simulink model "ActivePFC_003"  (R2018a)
settings: Solver=FixedStepDiscrete  StartTime=0.0  StopTime=inf  RelTol=1e-3  EnableMultiTasking=on
model workspace (MAT data in the model file):
  VoRef = 700
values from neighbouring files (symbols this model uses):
  Tcontrol = 5e-5    (= 5e-05)    [Sample_Time.m]
  Tmeasure = 5e-5     *2    (= 0.0001)    [Sample_Time.m]
  Tsample = 1e-6    (= 1e-06)    [Sample_Time.m]
  Tscope = Tcontrol*20    (= 0.001)    [Sample_Time.m]
undefined symbols (not defined in the file or in its folder): A, ADCIN0, ADCIN1, ADCINA0, ADCINB0, bit, Compare, Control, controller, conversion, DCAEVT1, DCAEVT1FILT, Digital, DiscIntNeverNeededParam, ended, Event, Filtered, GPTRIP1SEL, GPTRIP2SEL, input, Module, of, PI, PWM_Library, Single, start, Trip, TZ1, TZ2, version, Zone
libraries: c2837xDlib x23, c2802xlib x5, simulink x3, simulink_extras x2

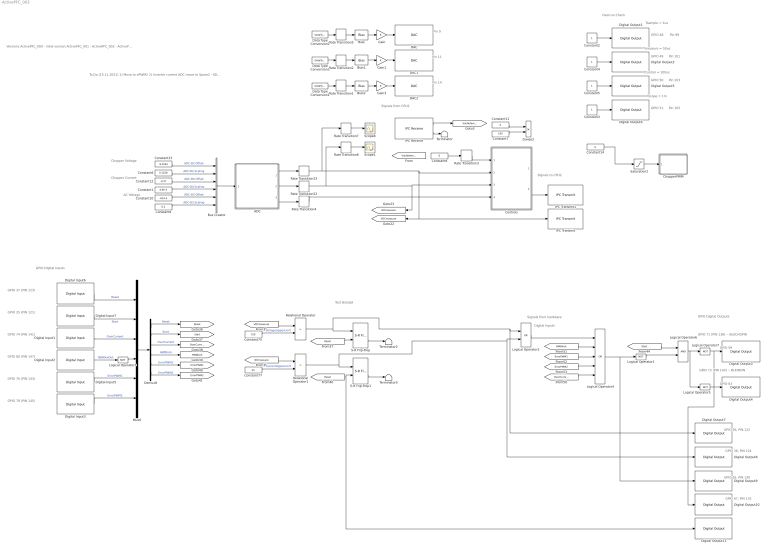
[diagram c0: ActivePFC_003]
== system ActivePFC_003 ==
  note: Test Bistabil
  note: GPIO 38, PIN 124
  note: GPIO 36, PIN 122
  note: GPIO 35 (PIN 121)
  note: GPIO 59
  note: GPIO 63
  note: GPIO Digital Inputs
  note: Digital Inputs
  note: GPIO 74 (PIN 141)
  note: GPIO Digital Outputs
  note: GPIO 80 (PIN 147)
  note: GPIO 37 (PIN 123)
  note: GPIO 78 (PIN 145)
  note: Signals to CPU2
  note: GPIO 73 (PIN 140) -- BLKINVIN
  note: GPIO 76 (PIN 143)
  note: GPIO 71 (PIN 138) -- BLKCHOPIN
  note: Signals from hardware
  note: GPIO 49
  note: Overrun Check
  note: Tcontrol = 100us
  note: Pin 105
  note: Pin 99
  note: Tmeasure = 50us
  note: GPIO 50
  note: GPIO 48
  note: Pin 101
  note: GPIO 51
  note: Pin 103
  note: Tsample = 1us
  note: Tscope = 1m
  note: GPIO 67, PIN 132
  note: GPIO 65, PIN 130
  note: Chopper Current
  note: AC Voltage
  note: Chopper Voltage
  note: Pin 11
  note: Pin 14
  note: Pin 9
  note: Versions ActivePFC_000 - inital version ActivePFC_001 - ActivePFC_002 - ActivePFC_003 - current version ActivePFC_004 - future version
  note: To Do (15.11.2021) 1) Move to ePWM2 2) Inverter current ADC move to Spare2 - ADC-B5 (Pin 26) 3) Change PCB resistor to 100 Ohm for Spare2 4) Check scaling for Spare2
  note: Signals from CPU2
  ADC : Subsystem
  Bias : Bias  Commented=on  Bias=0.0
  Bias1 : Bias  Commented=on  Bias=0.0
  Bias2 : Bias  Commented=on  Bias=0.0
  Bus Creator : BusCreator  Inputs=6
  ChopperPWM : Subsystem
  Constant1 : Constant  Value=4.9e-3  OutDataTypeStr=single  SampleTime=0.1
  Constant10 : Constant  Value=-614.4  OutDataTypeStr=single  SampleTime=0.1
  Constant11 : Constant  Value=0  OutDataTypeStr=single  SampleTime=Tcontrol
  Constant12 : Constant  Value=-0.27  OutDataTypeStr=single  SampleTime=0.1
  Constant13 : Constant  Value=-9.2581  OutDataTypeStr=single  SampleTime=0.1
  Constant14 : Constant  Value=0  OutDataTypeStr=single  SampleTime=Tcontrol
  Constant2 : Constant  Commented=on  SampleTime=Tsample
  Constant3 : Constant  SampleTime=Tscope
  Constant4 : Constant  SampleTime=Tmeasure
  Constant5 : Constant  SampleTime=Tcontrol
  Constant6 : Constant  Value=0.1228  OutDataTypeStr=single  SampleTime=0.1
  Constant7 : Constant  Value=100  OutDataTypeStr=single  SampleTime=Tcontrol
  Constant75 : Constant  Value=750  OutDataTypeStr=single  SampleTime=Tcontrol
  Constant77 : Constant  Value=20  OutDataTypeStr=single  SampleTime=Tcontrol
  Constant8 : Constant  Value=0  OutDataTypeStr=single  SampleTime=Tcontrol
  Constant9 : Constant  Value=0.3  OutDataTypeStr=single  SampleTime=0.1
  Controls : Subsystem
  DAC : c2837xDlib/DAC  Commented=on  channel=A  saturate=off
  DAC1 : c2837xDlib/DAC  Commented=on  channel=B  saturate=off
  DAC2 : c2837xDlib/DAC  Commented=on  channel=C  saturate=off
  Data Type Conversion1 : DataTypeConversion  Commented=on  OutDataTypeStr=single
  Data Type Conversion2 : DataTypeConversion  Commented=on  OutDataTypeStr=single
  Data Type Conversion3 : DataTypeConversion  Commented=on  OutDataTypeStr=single
  Demux8 : Demux  Outputs=6
  Digital Input1 : c2837xDlib/Digital Input  GPIO_Number=GPIO72~GPIO79  GPIO_Bit0=off  GPIO_Bit1=off  GPIO_Bit2=on  GPIO_Bit3=off  GPIO_Bit4=off  GPIO_Bit5=off  GPIO_Bit6=off  GPIO_Bit7=off  sampleTime=Tcontrol  dataType=auto  GPIO_Bit0_Qualification=Sync to SYSCLKOUT  GPIO_Bit1_Qualification=Sync to SYSCLKOUT  GPIO_Bit2_Qualification=Sync to SYSCLKOUT  GPIO_Bit3_Qualification=Sync to SYSCLKOUT  GPIO_Bit4_Qualification=Sync to SYSCLKOUT  GPIO_Bit5_Qualification=Sync to SYSCLKOUT  GPIO_Bit6_Qualification=Sync to SYSCLKOUT  GPIO_Bit7_Qualification=Sync to SYSCLKOUT  Qualification_Period=-1
  Digital Input2 : c2837xDlib/Digital Input  GPIO_Number=GPIO80~GPIO87  GPIO_Bit0=on  GPIO_Bit1=off  GPIO_Bit2=off  GPIO_Bit3=off  GPIO_Bit4=off  GPIO_Bit5=off  GPIO_Bit6=off  GPIO_Bit7=off  sampleTime=Tcontrol  dataType=auto  GPIO_Bit0_Qualification=Sync to SYSCLKOUT  GPIO_Bit1_Qualification=Sync to SYSCLKOUT  GPIO_Bit2_Qualification=Sync to SYSCLKOUT  GPIO_Bit3_Qualification=Sync to SYSCLKOUT  GPIO_Bit4_Qualification=Sync to SYSCLKOUT  GPIO_Bit5_Qualification=Sync to SYSCLKOUT  GPIO_Bit6_Qualification=Sync to SYSCLKOUT  GPIO_Bit7_Qualification=Sync to SYSCLKOUT  Qualification_Period=-1
  Digital Input3 : c2837xDlib/Digital Input  GPIO_Number=GPIO72~GPIO79  GPIO_Bit0=off  GPIO_Bit1=off  GPIO_Bit2=off  GPIO_Bit3=off  GPIO_Bit4=off  GPIO_Bit5=off  GPIO_Bit6=on  GPIO_Bit7=off  sampleTime=Tcontrol  dataType=auto  GPIO_Bit0_Qualification=Sync to SYSCLKOUT  GPIO_Bit1_Qualification=Sync to SYSCLKOUT  GPIO_Bit2_Qualification=Sync to SYSCLKOUT  GPIO_Bit3_Qualification=Sync to SYSCLKOUT  GPIO_Bit4_Qualification=Sync to SYSCLKOUT  GPIO_Bit5_Qualification=Sync to SYSCLKOUT  GPIO_Bit6_Qualification=Sync to SYSCLKOUT  GPIO_Bit7_Qualification=Sync to SYSCLKOUT  Qualification_Period=-1
  Digital Input5 : c2837xDlib/Digital Input  GPIO_Number=GPIO72~GPIO79  GPIO_Bit0=off  GPIO_Bit1=off  GPIO_Bit2=off  GPIO_Bit3=off  GPIO_Bit4=on  GPIO_Bit5=off  GPIO_Bit6=off  GPIO_Bit7=off  sampleTime=Tcontrol  dataType=auto  GPIO_Bit0_Qualification=Sync to SYSCLKOUT  GPIO_Bit1_Qualification=Sync to SYSCLKOUT  GPIO_Bit2_Qualification=Sync to SYSCLKOUT  GPIO_Bit3_Qualification=Sync to SYSCLKOUT  GPIO_Bit4_Qualification=Sync to SYSCLKOUT  GPIO_Bit5_Qualification=Sync to SYSCLKOUT  GPIO_Bit6_Qualification=Sync to SYSCLKOUT  GPIO_Bit7_Qualification=Sync to SYSCLKOUT  Qualification_Period=-1
  Digital Input6 : c2837xDlib/Digital Input  GPIO_Number=GPIO32~GPIO39  GPIO_Bit0=off  GPIO_Bit1=off  GPIO_Bit2=off  GPIO_Bit3=off  GPIO_Bit4=off  GPIO_Bit5=on  GPIO_Bit6=off  GPIO_Bit7=off  sampleTime=Tcontrol  dataType=auto  GPIO_Bit0_Qualification=Sync to SYSCLKOUT  GPIO_Bit1_Qualification=Sync to SYSCLKOUT  GPIO_Bit2_Qualification=Sync to SYSCLKOUT  GPIO_Bit3_Qualification=Sync to SYSCLKOUT  GPIO_Bit4_Qualification=Sync to SYSCLKOUT  GPIO_Bit5_Qualification=Sync to SYSCLKOUT  GPIO_Bit6_Qualification=Sync to SYSCLKOUT  GPIO_Bit7_Qualification=Sync to SYSCLKOUT  Qualification_Period=-1
  Digital Input7 : c2837xDlib/Digital Input  GPIO_Number=GPIO32~GPIO39  GPIO_Bit0=off  GPIO_Bit1=off  GPIO_Bit2=off  GPIO_Bit3=on  GPIO_Bit4=off  GPIO_Bit5=off  GPIO_Bit6=off  GPIO_Bit7=off  sampleTime=Tcontrol  dataType=auto  GPIO_Bit0_Qualification=Sync to SYSCLKOUT  GPIO_Bit1_Qualification=Sync to SYSCLKOUT  GPIO_Bit2_Qualification=Sync to SYSCLKOUT  GPIO_Bit3_Qualification=Sync to SYSCLKOUT  GPIO_Bit4_Qualification=Sync to SYSCLKOUT  GPIO_Bit5_Qualification=Sync to SYSCLKOUT  GPIO_Bit6_Qualification=Sync to SYSCLKOUT  GPIO_Bit7_Qualification=Sync to SYSCLKOUT  Qualification_Period=-1
  Digital Output1 : c2837xDlib/Digital Output  Commented=on  GPIO_Number=GPIO48~GPIO55  GPIO_Bit0=on  GPIO_BIT0_Toggle=on  GPIO_Bit1=off  GPIO_BIT1_Toggle=off  GPIO_Bit2=off  GPIO_BIT2_Toggle=on  GPIO_Bit3=off  GPIO_BIT3_Toggle=off  GPIO_Bit4=off  GPIO_BIT4_Toggle=off  GPIO_Bit5=off  GPIO_BIT5_Toggle=off  GPIO_Bit6=off  GPIO_BIT6_Toggle=off  GPIO_Bit7=off  GPIO_BIT7_Toggle=off
  Digital Output10 : c2837xDlib/Digital Output  GPIO_Number=GPIO64~GPIO71  GPIO_Bit0=off  GPIO_BIT0_Toggle=off  GPIO_Bit1=off  GPIO_BIT1_Toggle=off  GPIO_Bit2=off  GPIO_BIT2_Toggle=off  GPIO_Bit3=on  GPIO_BIT3_Toggle=off  GPIO_Bit4=off  GPIO_BIT4_Toggle=off  GPIO_Bit5=off  GPIO_BIT5_Toggle=off  GPIO_Bit6=off  GPIO_BIT6_Toggle=off  GPIO_Bit7=off  GPIO_BIT7_Toggle=off
  Digital Output11 : c2837xDlib/Digital Output  GPIO_Number=GPIO64~GPIO71  GPIO_Bit0=off  GPIO_BIT0_Toggle=off  GPIO_Bit1=off  GPIO_BIT1_Toggle=off  GPIO_Bit2=off  GPIO_BIT2_Toggle=off  GPIO_Bit3=off  GPIO_BIT3_Toggle=off  GPIO_Bit4=off  GPIO_BIT4_Toggle=off  GPIO_Bit5=on  GPIO_BIT5_Toggle=off  GPIO_Bit6=off  GPIO_BIT6_Toggle=off  GPIO_Bit7=off  GPIO_BIT7_Toggle=off
  Digital Output2 : c2837xDlib/Digital Output  GPIO_Number=GPIO48~GPIO55  GPIO_Bit0=off  GPIO_BIT0_Toggle=on  GPIO_Bit1=on  GPIO_BIT1_Toggle=on  GPIO_Bit2=off  GPIO_BIT2_Toggle=on  GPIO_Bit3=off  GPIO_BIT3_Toggle=off  GPIO_Bit4=off  GPIO_BIT4_Toggle=off  GPIO_Bit5=off  GPIO_BIT5_Toggle=off  GPIO_Bit6=off  GPIO_BIT6_Toggle=off  GPIO_Bit7=off  GPIO_BIT7_Toggle=off
  Digital Output3 : c2837xDlib/Digital Output  GPIO_Number=GPIO64~GPIO71  GPIO_Bit0=off  GPIO_BIT0_Toggle=off  GPIO_Bit1=off  GPIO_BIT1_Toggle=off  GPIO_Bit2=off  GPIO_BIT2_Toggle=off  GPIO_Bit3=off  GPIO_BIT3_Toggle=off  GPIO_Bit4=off  GPIO_BIT4_Toggle=off  GPIO_Bit5=off  GPIO_BIT5_Toggle=off  GPIO_Bit6=off  GPIO_BIT6_Toggle=off  GPIO_Bit7=on  GPIO_BIT7_Toggle=off
  Digital Output4 : c2837xDlib/Digital Output  GPIO_Number=GPIO72~GPIO79  GPIO_Bit0=off  GPIO_BIT0_Toggle=off  GPIO_Bit1=on  GPIO_BIT1_Toggle=off  GPIO_Bit2=off  GPIO_BIT2_Toggle=off  GPIO_Bit3=off  GPIO_BIT3_Toggle=off  GPIO_Bit4=off  GPIO_BIT4_Toggle=off  GPIO_Bit5=off  GPIO_BIT5_Toggle=off  GPIO_Bit6=off  GPIO_BIT6_Toggle=off  GPIO_Bit7=off  GPIO_BIT7_Toggle=off
  Digital Output5 : c2837xDlib/Digital Output  GPIO_Number=GPIO48~GPIO55  GPIO_Bit0=off  GPIO_BIT0_Toggle=off  GPIO_Bit1=off  GPIO_BIT1_Toggle=off  GPIO_Bit2=on  GPIO_BIT2_Toggle=on  GPIO_Bit3=off  GPIO_BIT3_Toggle=off  GPIO_Bit4=off  GPIO_BIT4_Toggle=off  GPIO_Bit5=off  GPIO_BIT5_Toggle=off  GPIO_Bit6=off  GPIO_BIT6_Toggle=off  GPIO_Bit7=off  GPIO_BIT7_Toggle=off
  Digital Output6 : c2837xDlib/Digital Output  GPIO_Number=GPIO48~GPIO55  GPIO_Bit0=off  GPIO_BIT0_Toggle=on  GPIO_Bit1=off  GPIO_BIT1_Toggle=off  GPIO_Bit2=off  GPIO_BIT2_Toggle=on  GPIO_Bit3=on  GPIO_BIT3_Toggle=on  GPIO_Bit4=off  GPIO_BIT4_Toggle=off  GPIO_Bit5=off  GPIO_BIT5_Toggle=off  GPIO_Bit6=off  GPIO_BIT6_Toggle=off  GPIO_Bit7=off  GPIO_BIT7_Toggle=off
  Digital Output7 : c2837xDlib/Digital Output  GPIO_Number=GPIO32~GPIO39  GPIO_Bit0=off  GPIO_BIT0_Toggle=off  GPIO_Bit1=off  GPIO_BIT1_Toggle=off  GPIO_Bit2=off  GPIO_BIT2_Toggle=off  GPIO_Bit3=off  GPIO_BIT3_Toggle=off  GPIO_Bit4=on  GPIO_BIT4_Toggle=off  GPIO_Bit5=off  GPIO_BIT5_Toggle=off  GPIO_Bit6=off  GPIO_BIT6_Toggle=off  GPIO_Bit7=off  GPIO_BIT7_Toggle=off
  Digital Output8 : c2837xDlib/Digital Output  GPIO_Number=GPIO32~GPIO39  GPIO_Bit0=off  GPIO_BIT0_Toggle=off  GPIO_Bit1=off  GPIO_BIT1_Toggle=off  GPIO_Bit2=off  GPIO_BIT2_Toggle=off  GPIO_Bit3=off  GPIO_BIT3_Toggle=off  GPIO_Bit4=off  GPIO_BIT4_Toggle=off  GPIO_Bit5=off  GPIO_BIT5_Toggle=off  GPIO_Bit6=on  GPIO_BIT6_Toggle=off  GPIO_Bit7=off  GPIO_BIT7_Toggle=off
  Digital Output9 : c2837xDlib/Digital Output  GPIO_Number=GPIO64~GPIO71  GPIO_Bit0=off  GPIO_BIT0_Toggle=off  GPIO_Bit1=on  GPIO_BIT1_Toggle=off  GPIO_Bit2=off  GPIO_BIT2_Toggle=off  GPIO_Bit3=off  GPIO_BIT3_Toggle=off  GPIO_Bit4=off  GPIO_BIT4_Toggle=off  GPIO_Bit5=off  GPIO_BIT5_Toggle=off  GPIO_Bit6=off  GPIO_BIT6_Toggle=off  GPIO_Bit7=off  GPIO_BIT7_Toggle=off
  Divide2 : Product  Inputs=*/
  Gain : Gain  Commented=on
  Gain1 : Gain  Commented=on
  Gain3 : Gain  Commented=on
  IPC Receive : c2837xDlib/IPC Receive  SelectChannel=1  DataType=single  DataLength=1  EnableBlocking=off  SampleTime=Tcontrol
  IPC Transmit : c2837xDlib/IPC Transmit  SelectChannel=0  EnableBlocking=off
  IPC Transmit1 : c2837xDlib/IPC Transmit  SelectChannel=2  EnableBlocking=off
  Logical Operator{1,3,5,7} (4 alike) : Logic  Operator=NOT  AllPortsSameDT=off  OutDataTypeStr=boolean
  Logical Operator2 : Logic  Operator=OR  AllPortsSameDT=off  OutDataTypeStr=boolean
  Logical Operator4 : Logic  Operator=OR  Inputs=5  AllPortsSameDT=off  OutDataTypeStr=boolean
  Logical Operator6 : Logic  AllPortsSameDT=off  OutDataTypeStr=boolean
  Mux6 : Mux  Inputs=6
  Rate Transition1 : RateTransition  Commented=on  OutPortSampleTime=Tcontrol
  Rate Transition2 : RateTransition  Commented=on  OutPortSampleTime=Tcontrol
  Rate Transition{3..4,22..23} (4 alike) : RateTransition  OutPortSampleTime=Tcontrol
  Rate Transition5 : RateTransition  Commented=on  OutPortSampleTime=Tcontrol
  Rate Transition7 : RateTransition  OutPortSampleTime=Tscope
  Rate Transition8 : RateTransition  OutPortSampleTime=Tscope
  Relational Operator : RelationalOperator  Operator=>  OutDataTypeStr=boolean
  Relational Operator1 : RelationalOperator  Operator=>  OutDataTypeStr=boolean
  S-R Flip-Flop : simulink_extras/Flip Flops/S-R Flip-Flop  Commented=on  initial_condition=0
  S-R Flip-Flop1 : simulink_extras/Flip Flops/S-R Flip-Flop  Commented=on  initial_condition=0
  Saturation2 : Saturate  UpperLimit=0.98  LowerLimit=0
  Scope1 : Scope
  Scope8 : Scope
  Terminator : Terminator
  Terminator2 : Terminator
  Terminator5 : Terminator
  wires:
  Logical Operator4/1 -> Digital Output9/1, Logical Operator1/1
  Digital Input6/1 -> Mux6/1  "Reset"
  Digital Input7/1 -> Mux6/2  "Start"
  [Start] -> Logical Operator6/1
  Constant14/1 -> Saturation2/1
  Mux6/1 -> Demux8/1
  Digital Input1/1 -> Mux6/3  "OverCurrent"
  Constant11/1 -> Divide2/1
  ADC/1(ADC-B2) -> Rate Transition23/1
  [ErrorPWM1] -> Logical Operator4/3
  Relational Operator1/1 -> Digital Output8/1, Logical Operator2/2, S-R Flip-Flop1/1
  Constant77/1 -> Relational Operator1/2  "CurrentUpperLimit"
  [Reset] -> Digital Output11/1, S-R Flip-Flop1/2
  Relational Operator/1 -> Digital Output7/1, Logical Operator2/1, S-R Flip-Flop/1
  [ErrorPWM2] -> Logical Operator4/4
  [IDCmeasure] -> Relational Operator1/1
  [HWBlock] -> Logical Operator4/2
  Digital Input3/1 -> Mux6/6  "ErrorPWM2"
  Logical Operator2/1 -> Logical Operator4/1
  Demux8/6 -> [ErrorPWM2]  "ErrorPWM2"
  Constant7/1 -> Divide2/2
  S-R Flip-Flop1/2 -> Terminator5/1
  [Reset] -> S-R Flip-Flop/2
  Demux8/3 -> [OverCurrent]  "OverCurrent"
  Demux8/2 -> [Start]  "Start"
  [VDCmeasure] -> Relational Operator/1
  Demux8/1 -> [Reset]  "Reset"
  Demux8/5 -> [ErrorPWM1]  "ErrorPWM1"
  Demux8/4 -> [HWBlock]  "HWBlock"
  ADC/2(ADC-B4) -> Rate Transition22/1
  S-R Flip-Flop/2 -> Terminator2/1
  Saturation2/1 -> ChopperPWM/1(PWM)
  Digital Input5/1 -> Mux6/5  "ErrorPWM1"
  [OverCurrent] -> Logical Operator4/5
  Constant75/1 -> Relational Operator/2  "VoltageUpperLimit"
  Digital Input2/1 -> Logical Operator3/1  "NBlkHwOut"
  Rate Transition22/1 -> Rate Transition8/1, Controls/3(Inductor Current), [IDCmeasure]
  Rate Transition7/1 -> Scope8/1
  Constant2/1 -> Digital Output1/1
  Constant4/1 -> Digital Output2/1
  Constant3/1 -> Digital Output6/1
  Constant5/1 -> Digital Output5/1
  Rate Transition23/1 -> Rate Transition7/1, Controls/2(Output Voltage), [VDCmeasure], IPC Transmit/1
  Logical Operator6/1 -> Logical Operator5/1, Logical Operator7/1
  Logical Operator5/1 -> Digital Output4/1
  Logical Operator7/1 -> Digital Output10/1, Digital Output3/1
  Logical Operator1/1 -> Logical Operator6/2
  Logical Operator3/1 -> Mux6/4
  Rate Transition3/1 -> Controls/1(VoRef)
  ADC/3(ADC-B3) -> Rate Transition4/1
  Constant8/1 -> Rate Transition3/1
  Rate Transition4/1 -> Controls/4(Source Voltage)
  Constant10/1 -> Bus Creator/5  "ADC-B3 Offset"
  Constant9/1 -> Bus Creator/6  "ADC-B3 Scaling"
  Constant12/1 -> Bus Creator/3  "ADC-B4 Offset"
  Constant13/1 -> Bus Creator/1  "ADC-B2 Offset"
  Constant1/1 -> Bus Creator/4  "ADC-B4 Scaling"
  Bus Creator/1 -> ADC/1(Scaling and Offset)
  Rate Transition8/1 -> Scope1/1
  Constant6/1 -> Bus Creator/2  "ADC-B2 Scaling"
  Rate Transition2/1 -> Bias1/1
  Data Type Conversion1/1 -> Rate Transition1/1
  Data Type Conversion3/1 -> Rate Transition2/1
  Rate Transition1/1 -> Bias2/1
  Rate Transition5/1 -> Bias/1
  Data Type Conversion2/1 -> Rate Transition5/1
  Gain/1 -> DAC/1
  Gain1/1 -> DAC1/1
  Gain3/1 -> DAC2/1
  Bias/1 -> Gain/1
  Bias1/1 -> Gain1/1
  Bias2/1 -> Gain3/1
  Controls/2(Angle) -> IPC Transmit1/1
  IPC Receive/1 -> [VdcReference]
  IPC Receive/2 -> Terminator/1

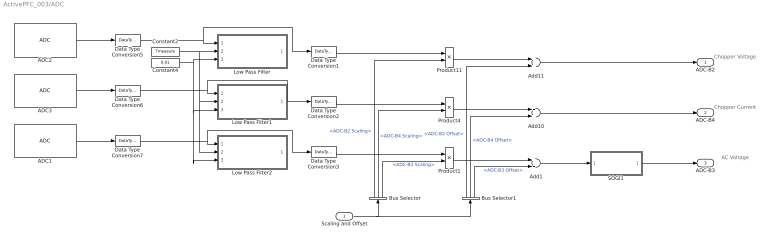
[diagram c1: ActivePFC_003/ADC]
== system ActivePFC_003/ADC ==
  note: Chopper Voltage
  note: Chopper Current
  note: AC Voltage
  Scaling and Offset : Inport
  ADC1 : c2802xlib/ADC  blkParamProc=C2000_Type4  ADCModule=B  samplingMode=Single sample mode  ADCResolution=12-bit (Single-ended input)  useSOC1=SOC1  useSOC2=SOC0_SOC1  SOCAcquisitionWindow=15  SOCTriggerSource=Software  SOCInterruptTrigger=ADCINT2  Ts=Tmeasure  dType=single  postInterrupt=off  interruptSel=ADCINT1  ADCINTContinuous=on  endma=off  chdma=1  conv1=ADCINA0  conv2=ADCINA0 and ADCINB0  conv1_Type4=ADCIN3  conv2_Type4=ADCIN0 and ADCIN1
  ADC2 : c2802xlib/ADC  blkParamProc=C2000_Type4  ADCModule=B  samplingMode=Single sample mode  ADCResolution=12-bit (Single-ended input)  useSOC1=SOC0  useSOC2=SOC0_SOC1  SOCAcquisitionWindow=15  SOCTriggerSource=Software  SOCInterruptTrigger=ADCINT2  Ts=Tmeasure  dType=single  postInterrupt=off  interruptSel=ADCINT1  ADCINTContinuous=on  endma=off  chdma=1  conv1=ADCINA0  conv2=ADCINA0 and ADCINB0  conv1_Type4=ADCIN2  conv2_Type4=ADCIN0 and ADCIN1
  ADC3 : c2802xlib/ADC  blkParamProc=C2000_Type4  ADCModule=B  samplingMode=Single sample mode  ADCResolution=12-bit (Single-ended input)  useSOC1=SOC2  useSOC2=SOC0_SOC1  SOCAcquisitionWindow=15  SOCTriggerSource=Software  SOCInterruptTrigger=ADCINT2  Ts=Tmeasure  dType=single  postInterrupt=off  interruptSel=ADCINT1  ADCINTContinuous=on  endma=off  chdma=1  conv1=ADCINA0  conv2=ADCINA0 and ADCINB0  conv1_Type4=ADCIN4  conv2_Type4=ADCIN0 and ADCIN1
  Add1 : Sum  OutDataTypeStr=single
  Add10 : Sum  OutDataTypeStr=single
  Add11 : Sum  OutDataTypeStr=single
  Bus Selector : BusSelector  OutputSignals=ADC-B2 Scaling,ADC-B4 Scaling,ADC-B3 Scaling
  Bus Selector1 : BusSelector  OutputSignals=ADC-B2 Offset,ADC-B4 Offset,ADC-B3 Offset
  Constant2 : Constant  Value=Tmeasure
  Constant4 : Constant  Value=0.01
  Data Type Conversion1 : DataTypeConversion  OutDataTypeStr=single
  Data Type Conversion2 : DataTypeConversion  OutDataTypeStr=single
  Data Type Conversion3 : DataTypeConversion  OutDataTypeStr=single
  Data Type Conversion5 : DataTypeConversion  OutDataTypeStr=double
  Data Type Conversion6 : DataTypeConversion  OutDataTypeStr=double
  Data Type Conversion7 : DataTypeConversion  OutDataTypeStr=double
  Low Pass Filter : Subsystem  Commented=on
      mask help: <!DOCTYPE HTML PUBLIC "-//W3C//DTD HTML 4.01 Transitional//EN"> <html><head> </head> <body> <p style="text-align: center; font-weight: bold;">Low Pass Filter </p> <p><strong>Inputs: </strong></p> <ol> <li>Input (single)</li> <li>Sample Time (single)</li> <li>Time Constant (single)</li> </ol> <p><strong>Outputs: </strong></p> <ol> <li>Output (single)</li> </ol> </body></html>
  Low Pass Filter1 : Subsystem  Commented=on
      mask help: <!DOCTYPE HTML PUBLIC "-//W3C//DTD HTML 4.01 Transitional//EN"> <html><head> </head> <body> <p style="text-align: center; font-weight: bold;">Low Pass Filter </p> <p><strong>Inputs: </strong></p> <ol> <li>Input (single)</li> <li>Sample Time (single)</li> <li>Time Constant (single)</li> </ol> <p><strong>Outputs: </strong></p> <ol> <li>Output (single)</li> </ol> </body></html>
  Low Pass Filter2 : Subsystem  Commented=on
      mask help: <!DOCTYPE HTML PUBLIC "-//W3C//DTD HTML 4.01 Transitional//EN"> <html><head> </head> <body> <p style="text-align: center; font-weight: bold;">Low Pass Filter </p> <p><strong>Inputs: </strong></p> <ol> <li>Input (single)</li> <li>Sample Time (single)</li> <li>Time Constant (single)</li> </ol> <p><strong>Outputs: </strong></p> <ol> <li>Output (single)</li> </ol> </body></html>
  Product1 : Product  OutDataTypeStr=single
  Product11 : Product  OutDataTypeStr=single
  Product4 : Product  OutDataTypeStr=single
  SOGI1 : Subsystem  TreatAsAtomicUnit=on  mask{Freq=50, SampleTime=Tcontrol, UpperLimit=1000, LowerLimit=-1000}
      mask prompts: Freq "Frequency, Hz"; SampleTime "Sample Time, s"; UpperLimit "Upper Limit"; LowerLimit "Lower Limit"
  ADC-B2 : Outport
  ADC-B4 : Outport  Port=2
  ADC-B3 : Outport  Port=3
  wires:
  Bus Selector/2 -> Product4/2  "<ADC-B4 Scaling>"
  Bus Selector/3 -> Product1/2  "<ADC-B3 Scaling>"
  Scaling and Offset/1 -> Bus Selector/1, Bus Selector1/1
  Bus Selector/1 -> Product11/2  "<ADC-B2 Scaling>"
  Product11/1 -> Add11/1
  Product4/1 -> Add10/1
  Product1/1 -> Add1/1
  Add1/1 -> SOGI1/1(In)
  Add10/1 -> ADC-B4/1
  Add11/1 -> ADC-B2/1
  SOGI1/1(Out) -> ADC-B3/1
  Constant4/1 -> Low Pass Filter2/3(TimeConstant), Low Pass Filter1/3(TimeConstant), Low Pass Filter/3(TimeConstant)
  Constant2/1 -> Low Pass Filter2/2(SamplePeriod), Low Pass Filter1/2(SamplePeriod), Low Pass Filter/2(SamplePeriod)
  ADC1/1 -> Data Type Conversion7/1
  ADC3/1 -> Data Type Conversion6/1
  ADC2/1 -> Data Type Conversion5/1
  Data Type Conversion5/1 -> Data Type Conversion1/1, Low Pass Filter/1(Input)
  Data Type Conversion6/1 -> Data Type Conversion2/1, Low Pass Filter1/1(Input)
  Data Type Conversion7/1 -> Data Type Conversion3/1, Low Pass Filter2/1(Input)
  Data Type Conversion1/1 -> Product11/1
  Data Type Conversion2/1 -> Product4/1
  Data Type Conversion3/1 -> Product1/1
  Bus Selector1/3 -> Add1/2  "<ADC-B3 Offset>"
  Bus Selector1/2 -> Add10/2  "<ADC-B4 Offset>"
  Bus Selector1/1 -> Add11/2  "<ADC-B2 Offset>"

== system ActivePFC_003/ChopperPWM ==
  note: CMPA = (100 % - dut cycle) * (TBPRD + 1) - 1 TBPRD = f_TBCLK / f_PWM - 1
  PWM : Inport
  Add15 : Sum  Inputs=+-
  Constant1 : Constant  OutDataTypeStr=single  SampleTime=Tcontrol
  Constant16 : Constant  Value=5000  OutDataTypeStr=single  SampleTime=Tcontrol
  Data Type Conversion18 : DataTypeConversion  OutDataTypeStr=single
  Product22 : Product
  ePWM2 : c2802xlib/ePWM  useModule=ePWM1  ePWMxLINKTBPRD=Not Linked  periodUnits=Clock cycles  timerSource=Specify via dialog  timerPeriod_clk=4999  timerPeriod_sec=0.0001  tbshadow=Counter equals to zero  countingMode=Up  phaseActiveEnable=Disable  phaseDirection=Count down after sync  phaseActive=0  synchronizationEnable=off  dcaevt1Sync=off  dcbevt1Sync=off  synchronizationOption=Disable  clockPrescale=1  HSclockPrescale=1  enswap=off  ePWMxAStatus=on  ePWMxAactionLogic1=Set  ePWMxAactionLogic2=Clear  ePWMxAactionLogic3=Clear  ePWMxAactionLogic4=Set  ePWMxAactionLogic5=Do nothing  ePWMxAactionLogic6=Do nothing  ePWMxALoadMode=Load on counter equals to zero (CTR=Zero)  ePWMxACSFenable=off  ePWMxACSFvalue=Forcing disable  ePWMxASFreload=Zero  ePWMxBStatus=off  ePWMxBactionLogic1=Clear  ePWMxBactionLogic2=Set  ePWMxBactionLogic3=Do nothing  ePWMxBactionLogic4=Do nothing  ePWMxBactionLogic5=Set  ePWMxBactionLogic6=Clear  ePWMxBLoadMode=Load on counter equals to zero (CTR=Zero)  ePWMxBCSFenable=off  ePWMxBCSFvalue=Forcing disable  ePWMxBSFreload=Zero  ePWNxBOutWay=off  ePWMxLINKCMPA=Not Linked  CMPAUnits=Clock cycles  CMPASource=Input port  CMPAValue_per=50  CMPAValue_clk=3750  enCMPAshadow=Counter equals to zero  ePWMxLINKCMPB=Not Linked  CMPBUnits=Clock cycles  CMPBSource=Specify via dialog  CMPBValue_per=50  CMPBValue_clk=3750  enCMPBshadow=Counter equals to zero  ePWMxLINKCMPC=Not Linked  CMPCUnits=Clock cycles  CMPCSource=Specify via dialog  CMPCValue_per=50  CMPCValue_clk=32000  enCMPCshadow=Counter equals to zero  ePWMxLINKCMPD=Not Linked  CMPDUnits=Clock cycles  CMPDSource=Specify via dialog  CMPDValue_per=50  CMPDValue_clk=32000  enCMPDshadow=Counter equals to zero  enableDBePWMxA=off  enableDBePWMxB=off  enhalfcycle=off  DBpolarity=Active high complementary (AHC)  DBedgeDelay=Positive  DBSource_ePWMxA=ePWMxA  DBSource_ePWMxB=ePWMxA  DBperiodSource=Input port  REDperiod=0  FEDperiod=0  adcstartModuleA=off  adcrequestEventA=First event  adcstartEventA=Digital Compare Module A Event 1 start of conversion (DCAEVT1.soc)  adcstartEventA_type2=Digital Compare Module A Event 1 start of conversion (DCAEVT1.soc)  adcstartModuleB=off  adcrequestEventB=First event  adcstartEventB=Counter equals to zero (CTR=Zero)  adcstartEventB_type2=Counter equals to zero (CTR=Zero)  intEn=off  intPrd=First event  intSel=Counter equals to zero (CTR=Zero)  intSel_type2=Counter equals to zero (CTR=Zero)  hrpe=off  enHRPWM=off  HRPWM_LoadMode=Counter equals to period (CTR=PRD)  HRPWM_CTLMode=Duty or Period control mode  HRPWM_EDGMode=Both edge  hrpeb=off  enHRPWMB=off  HRPWM_LoadModeB=Counter equals to zero (CTR=ZERO)  HRPWM_CTLModeB=Duty or Period control mode  HRPWM_EDGModeB=Both edge  enSFO=on  enautoconv=on  chopperEnable=off  chopperFrequency=1  chopperFirstwidth=1  chopperDuty=12.5%  tripZonesource=Specify via dialog  tzselOSHT1=off  tzselOSHT2=off  tzselOSHT3=off  tzselOSHDCAEV1=off  tzselOSHDCBEV1=off  tzselCBC1=off  tzselCBC2=off  tzselCBC3=off  tzselCBCDCAEV2=off  tzselCBCDCBEV2=off  tzselOSHT4=off  tzselOSHT5=off  tzselOSHT6=off  tzselCBC4=off  tzselCBC5=off  tzselCBC6=off  enTzOstIntr=off  enTzCbcIntr=off  enTzDCAEVT1Intr=off  enTzDCAEVT2Intr=off  enTzDCBEVT1Intr=off  enTzDCBEVT2Intr=off  ePWMxAforced=No action  ePWMxBforced=No action  DCAEVT1forced=No action  DCBEVT1forced=No action  DCAEVT2forced=No action  DCBEVT2forced=No action  dcah=Trip Zone 1 input (TZ1)  dcal=Trip Zone 2 input (TZ2)  dcbh=Trip Zone 1 input (TZ1)  dcbl=Trip Zone 2 input (TZ2)  dcah_type2=GPTRIP1SEL/(TZ1)  dcal_type2=GPTRIP2SEL/(TZ2)  dcbh_type2=GPTRIP1SEL/(TZ1)  dcbl_type2=GPTRIP2SEL/(TZ2)  gendcaevt1=Event disabled  gendcaevt2=Event disabled  gendcbevt1=Event disabled  gendcbevt2=Event disabled  dcaevt1src=DCAEVT1 with sync  dcaevt2src=DCAEVT2 with sync  dcbevt1src=DCBEVT1 with sync  dcbevt2src=DCBEVT2 with sync  pulsesel=Counter equals to zero (CTR=Zero)  blankinv=off  blankoffset=0  blankwidth=0  evsrcsel=Filtered version of DCAEVT1 (DCAEVT1FILT)  encape=off  PwmType=C2000_Type4
  ePWM3 : c2802xlib/ePWM  Commented=on  useModule=ePWM2  ePWMxLINKTBPRD=Not Linked  periodUnits=Clock cycles  timerSource=Specify via dialog  timerPeriod_clk=4999  timerPeriod_sec=0.0001  tbshadow=Counter equals to zero  countingMode=Up  phaseActiveEnable=Disable  phaseDirection=Count down after sync  phaseActive=0  synchronizationEnable=off  dcaevt1Sync=off  dcbevt1Sync=off  synchronizationOption=Disable  clockPrescale=1  HSclockPrescale=1  enswap=off  ePWMxAStatus=on  ePWMxAactionLogic1=Set  ePWMxAactionLogic2=Clear  ePWMxAactionLogic3=Clear  ePWMxAactionLogic4=Set  ePWMxAactionLogic5=Do nothing  ePWMxAactionLogic6=Do nothing  ePWMxALoadMode=Load on counter equals to zero (CTR=Zero)  ePWMxACSFenable=off  ePWMxACSFvalue=Forcing disable  ePWMxASFreload=Zero  ePWMxBStatus=off  ePWMxBactionLogic1=Clear  ePWMxBactionLogic2=Set  ePWMxBactionLogic3=Do nothing  ePWMxBactionLogic4=Do nothing  ePWMxBactionLogic5=Set  ePWMxBactionLogic6=Clear  ePWMxBLoadMode=Load on counter equals to zero (CTR=Zero)  ePWMxBCSFenable=off  ePWMxBCSFvalue=Forcing disable  ePWMxBSFreload=Zero  ePWNxBOutWay=off  ePWMxLINKCMPA=Not Linked  CMPAUnits=Clock cycles  CMPASource=Input port  CMPAValue_per=50  CMPAValue_clk=3750  enCMPAshadow=Counter equals to zero  ePWMxLINKCMPB=Not Linked  CMPBUnits=Clock cycles  CMPBSource=Specify via dialog  CMPBValue_per=50  CMPBValue_clk=3750  enCMPBshadow=Counter equals to zero  ePWMxLINKCMPC=Not Linked  CMPCUnits=Clock cycles  CMPCSource=Specify via dialog  CMPCValue_per=50  CMPCValue_clk=32000  enCMPCshadow=Counter equals to zero  ePWMxLINKCMPD=Not Linked  CMPDUnits=Clock cycles  CMPDSource=Specify via dialog  CMPDValue_per=50  CMPDValue_clk=32000  enCMPDshadow=Counter equals to zero  enableDBePWMxA=off  enableDBePWMxB=off  enhalfcycle=off  DBpolarity=Active high complementary (AHC)  DBedgeDelay=Positive  DBSource_ePWMxA=ePWMxA  DBSource_ePWMxB=ePWMxA  DBperiodSource=Input port  REDperiod=0  FEDperiod=0  adcstartModuleA=off  adcrequestEventA=First event  adcstartEventA=Digital Compare Module A Event 1 start of conversion (DCAEVT1.soc)  adcstartEventA_type2=Digital Compare Module A Event 1 start of conversion (DCAEVT1.soc)  adcstartModuleB=off  adcrequestEventB=First event  adcstartEventB=Counter equals to zero (CTR=Zero)  adcstartEventB_type2=Counter equals to zero (CTR=Zero)  intEn=off  intPrd=First event  intSel=Counter equals to zero (CTR=Zero)  intSel_type2=Counter equals to zero (CTR=Zero)  hrpe=off  enHRPWM=off  HRPWM_LoadMode=Counter equals to period (CTR=PRD)  HRPWM_CTLMode=Duty or Period control mode  HRPWM_EDGMode=Both edge  hrpeb=off  enHRPWMB=off  HRPWM_LoadModeB=Counter equals to zero (CTR=ZERO)  HRPWM_CTLModeB=Duty or Period control mode  HRPWM_EDGModeB=Both edge  enSFO=on  enautoconv=on  chopperEnable=off  chopperFrequency=1  chopperFirstwidth=1  chopperDuty=12.5%  tripZonesource=Specify via dialog  tzselOSHT1=off  tzselOSHT2=off  tzselOSHT3=off  tzselOSHDCAEV1=off  tzselOSHDCBEV1=off  tzselCBC1=off  tzselCBC2=off  tzselCBC3=off  tzselCBCDCAEV2=off  tzselCBCDCBEV2=off  tzselOSHT4=off  tzselOSHT5=off  tzselOSHT6=off  tzselCBC4=off  tzselCBC5=off  tzselCBC6=off  enTzOstIntr=off  enTzCbcIntr=off  enTzDCAEVT1Intr=off  enTzDCAEVT2Intr=off  enTzDCBEVT1Intr=off  enTzDCBEVT2Intr=off  ePWMxAforced=No action  ePWMxBforced=No action  DCAEVT1forced=No action  DCBEVT1forced=No action  DCAEVT2forced=No action  DCBEVT2forced=No action  dcah=Trip Zone 1 input (TZ1)  dcal=Trip Zone 2 input (TZ2)  dcbh=Trip Zone 1 input (TZ1)  dcbl=Trip Zone 2 input (TZ2)  dcah_type2=GPTRIP1SEL/(TZ1)  dcal_type2=GPTRIP2SEL/(TZ2)  dcbh_type2=GPTRIP1SEL/(TZ1)  dcbl_type2=GPTRIP2SEL/(TZ2)  gendcaevt1=Event disabled  gendcaevt2=Event disabled  gendcbevt1=Event disabled  gendcbevt2=Event disabled  dcaevt1src=DCAEVT1 with sync  dcaevt2src=DCAEVT2 with sync  dcbevt1src=DCBEVT1 with sync  dcbevt2src=DCBEVT2 with sync  pulsesel=Counter equals to zero (CTR=Zero)  blankinv=off  blankoffset=0  blankwidth=0  evsrcsel=Filtered version of DCAEVT1 (DCAEVT1FILT)  encape=off  PwmType=C2000_Type4
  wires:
  PWM/1 -> Product22/1
  Product22/1 -> Add15/1
  Data Type Conversion18/1 -> ePWM3/1, ePWM2/1
  Constant16/1 -> Product22/2
  Constant1/1 -> Add15/2
  Add15/1 -> Data Type Conversion18/1

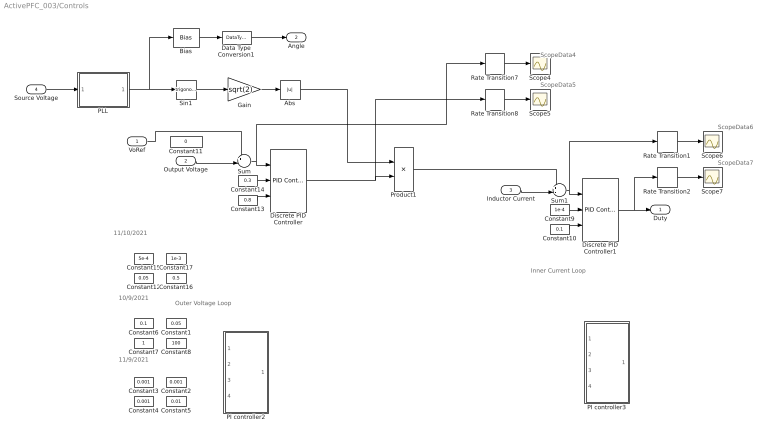
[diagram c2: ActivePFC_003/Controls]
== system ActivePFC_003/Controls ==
  note: ScopeData6
  note: ScopeData5
  note: ScopeData4
  note: 11/9/2021
  note: Inner Current Loop
  note: Outer Voltage Loop
  note: 10/9/2021
  note: ScopeData7
  note: 11/10/2021
  VoRef : Inport
  Output Voltage : Inport  Port=2
  Inductor Current : Inport  Port=3
  Source Voltage : Inport  Port=4
  Abs : Abs
  Bias : Bias  Commented=through  Bias=pi
  Constant1 : Constant  Value=0.05
  Constant10 : Constant  Value=0.1
  Constant11 : Constant  Value=0  OutDataTypeStr=single  SampleTime=Tcontrol
  Constant12 : Constant  Value=0.05
  Constant13 : Constant  Value=0.8
  Constant14 : Constant  Value=0.3
  Constant15 : Constant  Value=5e-4
  Constant16 : Constant  Value=0.5
  Constant17 : Constant  Value=1e-3
  Constant2 : Constant  Value=0.001
  Constant3 : Constant  Value=0.001
  Constant4 : Constant  Value=0.001
  Constant5 : Constant  Value=0.01
  Constant6 : Constant  Value=0.1
  Constant7 : Constant
  Constant8 : Constant  Value=100
  Constant9 : Constant  Value=1e-4
  Data Type Conversion1 : DataTypeConversion  OutDataTypeStr=single
  Discrete PID Controller : simulink/Continuous/PID Controller  Controller=PI  TimeDomain=Discrete-time  SampleTime=Tcontrol  IntegratorMethod=Backward Euler  FilterMethod=Forward Euler  Form=Parallel  UseFilter=on  ControllerParametersSource=external  P=1  I=1  D=0  N=100  InitialConditionSource=internal  InitialConditionForIntegrator=0  InitialConditionForFilter=0  ExternalReset=none  LimitOutput=on  UpperSaturationLimit=20  LowerSaturationLimit=-2  LinearizeAsGain=off  AntiWindupMode=clamping  Kb=1  TrackingMode=off  Kt=1  PParamMin=[]  PParamMax=[]  IParamMin=[]  IParamMax=[]  DParamMin=[]  DParamMax=[]  NParamMin=[]  NParamMax=[]  KbParamMin=[]  KbParamMax=[]  KtParamMin=[]  KtParamMax=[]  POutMin=[]  POutMax=[]  IOutMin=[]  IOutMax=[]  DOutMin=[]  DOutMax=[]  NOutMin=[]  NOutMax=[]  KbOutMin=[]  KbOutMax=[]  KtOutMin=[]  KtOutMax=[]  IntegratorOutMin=[]  IntegratorOutMax=[]  FilterOutMin=[]  FilterOutMax=[]  SumOutMin=[]  SumOutMax=[]  SumI1OutMin=[]  SumI1OutMax=[]  SumI2OutMin=[]  SumI2OutMax=[]  SumI3OutMin=[]  SumI3OutMax=[]  SumDOutMin=[]  SumDOutMax=[]  SaturationOutMin=[]  SaturationOutMax=[]  IntegratorContinuousStateAttributes=''  IntegratorStateMustResolveToSignalObject=off  IntegratorRTWStateStorageClass=Auto  FilterContinuousStateAttributes=''  FilterStateMustResolveToSignalObject=off  FilterRTWStateStorageClass=Auto  DifferentiatorICPrevScaledInput=0  DifferentiatorOutMin=[]  DifferentiatorOutMax=[]  FilterDiffOutCoefMin=[]  FilterDiffOutCoefMax=[]  SumDenOutMin=[]  SumDenOutMax=[]  SumNumOutMin=[]  SumNumOutMax=[]  ReciprocalOutMin=[]  ReciprocalOutMax=[]  DivideOutMin=[]  DivideOutMax=[]  TunerSelectOption=Transfer Function Based (PID Tuner App)
  Discrete PID Controller1 : simulink/Continuous/PID Controller  Controller=PI  TimeDomain=Discrete-time  SampleTime=Tcontrol  IntegratorMethod=Backward Euler  FilterMethod=Forward Euler  Form=Parallel  UseFilter=on  ControllerParametersSource=external  P=1  I=1  D=0  N=100  InitialConditionSource=internal  InitialConditionForIntegrator=0  InitialConditionForFilter=0  ExternalReset=none  LimitOutput=on  UpperSaturationLimit=0.98  LowerSaturationLimit=0  LinearizeAsGain=off  AntiWindupMode=clamping  Kb=1  TrackingMode=off  Kt=1  PParamMin=[]  PParamMax=[]  IParamMin=[]  IParamMax=[]  DParamMin=[]  DParamMax=[]  NParamMin=[]  NParamMax=[]  KbParamMin=[]  KbParamMax=[]  KtParamMin=[]  KtParamMax=[]  POutMin=[]  POutMax=[]  IOutMin=[]  IOutMax=[]  DOutMin=[]  DOutMax=[]  NOutMin=[]  NOutMax=[]  KbOutMin=[]  KbOutMax=[]  KtOutMin=[]  KtOutMax=[]  IntegratorOutMin=[]  IntegratorOutMax=[]  FilterOutMin=[]  FilterOutMax=[]  SumOutMin=[]  SumOutMax=[]  SumI1OutMin=[]  SumI1OutMax=[]  SumI2OutMin=[]  SumI2OutMax=[]  SumI3OutMin=[]  SumI3OutMax=[]  SumDOutMin=[]  SumDOutMax=[]  SaturationOutMin=[]  SaturationOutMax=[]  IntegratorContinuousStateAttributes=''  IntegratorStateMustResolveToSignalObject=off  IntegratorRTWStateStorageClass=Auto  FilterContinuousStateAttributes=''  FilterStateMustResolveToSignalObject=off  FilterRTWStateStorageClass=Auto  DifferentiatorICPrevScaledInput=0  DifferentiatorOutMin=[]  DifferentiatorOutMax=[]  FilterDiffOutCoefMin=[]  FilterDiffOutCoefMax=[]  SumDenOutMin=[]  SumDenOutMax=[]  SumNumOutMin=[]  SumNumOutMax=[]  ReciprocalOutMin=[]  ReciprocalOutMax=[]  DivideOutMin=[]  DivideOutMax=[]  TunerSelectOption=Transfer Function Based (PID Tuner App)
  Gain : Gain  Gain=sqrt(2)
  PI controller2 : Subsystem  Commented=on  AncestorBlock=PWM_Library/Control/PI controller  TreatAsAtomicUnit=on  mask(PI controller){SampleTime=Tcontrol, UpperLimit=20, LowerLimit=-2}
      mask prompts: SampleTime "Sample Time"; UpperLimit "Upper Limit"; LowerLimit "Lower Limit"
      mask help: PI controller
  PI controller3 : Subsystem  Commented=on  AncestorBlock=PWM_Library/Control/PI controller  TreatAsAtomicUnit=on  mask(PI controller){SampleTime=Tcontrol, UpperLimit=0.98, LowerLimit=0}
      mask prompts: SampleTime "Sample Time"; UpperLimit "Upper Limit"; LowerLimit "Lower Limit"
      mask help: PI controller
  PLL : Subsystem
  Product1 : Product
  Rate Transition{1..2,7..8} (4 alike) : RateTransition  OutPortSampleTime=Tscope
  Scope{4..7} (4 alike) : Scope
  Sin1 : Trigonometry
  Sum : Sum  Inputs=+-|
  Sum1 : Sum  Inputs=+-|
  Duty : Outport
  Angle : Outport  Port=2
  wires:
  PLL/1(Theta) -> Sin1/1, Bias/1
  Discrete PID Controller1/1 -> Rate Transition2/1, Duty/1
  Output Voltage/1 -> Sum/2
  Gain/1 -> Abs/1
  Sin1/1 -> Gain/1
  VoRef/1 -> Sum/1
  Product1/1 -> Sum1/1
  Source Voltage/1 -> PLL/1(In)
  Abs/1 -> Product1/1
  Bias/1 -> Data Type Conversion1/1
  Rate Transition7/1 -> Scope4/1
  Rate Transition8/1 -> Scope5/1
  Rate Transition1/1 -> Scope6/1
  Sum/1 -> Rate Transition7/1, Discrete PID Controller/1
  Constant14/1 -> Discrete PID Controller/2
  Constant13/1 -> Discrete PID Controller/3
  Constant10/1 -> Discrete PID Controller1/3
  Constant9/1 -> Discrete PID Controller1/2
  Inductor Current/1 -> Sum1/2
  Sum1/1 -> Rate Transition1/1, Discrete PID Controller1/1
  Discrete PID Controller/1 -> Rate Transition8/1, Product1/2
  Rate Transition2/1 -> Scope7/1
  Data Type Conversion1/1 -> Angle/1

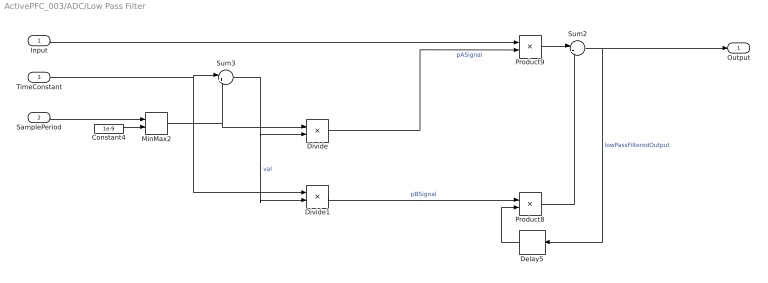
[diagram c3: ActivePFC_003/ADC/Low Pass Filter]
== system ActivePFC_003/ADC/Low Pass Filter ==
  Input : Inport
  SamplePeriod : Inport  Port=2
  TimeConstant : Inport  Port=3
  Constant4 : Constant  Value=1e-9  OutDataTypeStr=single
  Delay5 : Delay  DelayLength=1  InitialCondition=0
  Divide : Product  Inputs=*/
  Divide1 : Product  Inputs=*/
  MinMax2 : MinMax  Function=max  Inputs=2  OutDataTypeStr=single
  Product8 : Product  OutDataTypeStr=single
  Product9 : Product  OutDataTypeStr=single
  Sum2 : Sum  Inputs=|++  OutDataTypeStr=single
  Sum3 : Sum  Inputs=|++  OutDataTypeStr=single
  Output : Outport
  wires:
  SamplePeriod/1 -> MinMax2/1
  Constant4/1 -> MinMax2/2
  Input/1 -> Product9/1
  Delay5/1 -> Product8/2
  Divide1/1 -> Product8/1  "pBSignal"
  MinMax2/1 -> Divide/1, Sum3/2
  TimeConstant/1 -> Divide1/1, Sum3/1
  Product8/1 -> Sum2/2
  Product9/1 -> Sum2/1
  Divide/1 -> Product9/2  "pASignal"
  Sum2/1 -> Output/1, Delay5/1  "lowPassFilteredOutput"
  Sum3/1 -> Divide1/2, Divide/2  "val"

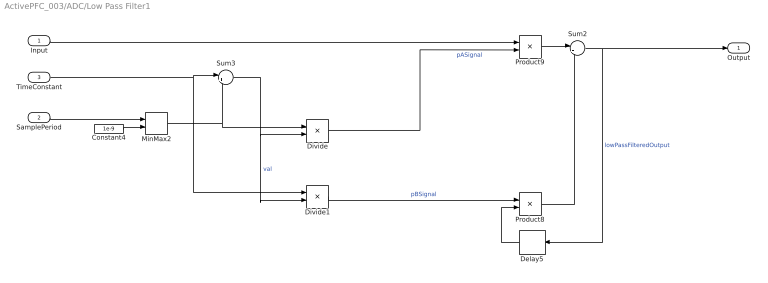
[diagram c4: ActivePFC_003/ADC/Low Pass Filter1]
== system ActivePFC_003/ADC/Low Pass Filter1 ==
  Input : Inport
  SamplePeriod : Inport  Port=2
  TimeConstant : Inport  Port=3
  Constant4 : Constant  Value=1e-9  OutDataTypeStr=single
  Delay5 : Delay  DelayLength=1  InitialCondition=0
  Divide : Product  Inputs=*/
  Divide1 : Product  Inputs=*/
  MinMax2 : MinMax  Function=max  Inputs=2  OutDataTypeStr=single
  Product8 : Product  OutDataTypeStr=single
  Product9 : Product  OutDataTypeStr=single
  Sum2 : Sum  Inputs=|++  OutDataTypeStr=single
  Sum3 : Sum  Inputs=|++  OutDataTypeStr=single
  Output : Outport
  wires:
  Sum3/1 -> Divide/2, Divide1/2  "val"
  Sum2/1 -> Delay5/1, Output/1  "lowPassFilteredOutput"
  Divide/1 -> Product9/2  "pASignal"
  Product9/1 -> Sum2/1
  Product8/1 -> Sum2/2
  TimeConstant/1 -> Sum3/1, Divide1/1
  MinMax2/1 -> Sum3/2, Divide/1
  Divide1/1 -> Product8/1  "pBSignal"
  Delay5/1 -> Product8/2
  Input/1 -> Product9/1
  Constant4/1 -> MinMax2/2
  SamplePeriod/1 -> MinMax2/1

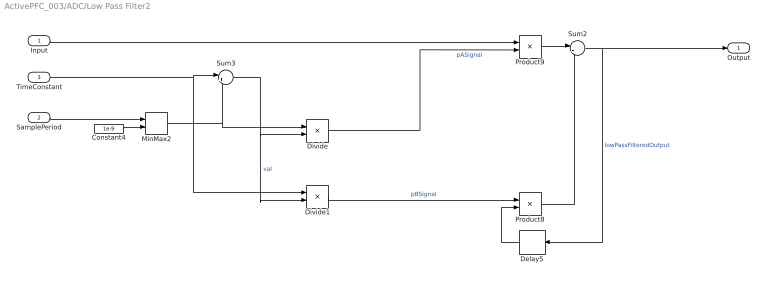
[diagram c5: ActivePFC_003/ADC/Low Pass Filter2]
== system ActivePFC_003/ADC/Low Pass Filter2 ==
  Input : Inport
  SamplePeriod : Inport  Port=2
  TimeConstant : Inport  Port=3
  Constant4 : Constant  Value=1e-9  OutDataTypeStr=single
  Delay5 : Delay  DelayLength=1  InitialCondition=0
  Divide : Product  Inputs=*/
  Divide1 : Product  Inputs=*/
  MinMax2 : MinMax  Function=max  Inputs=2  OutDataTypeStr=single
  Product8 : Product  OutDataTypeStr=single
  Product9 : Product  OutDataTypeStr=single
  Sum2 : Sum  Inputs=|++  OutDataTypeStr=single
  Sum3 : Sum  Inputs=|++  OutDataTypeStr=single
  Output : Outport
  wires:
  SamplePeriod/1 -> MinMax2/1
  Constant4/1 -> MinMax2/2
  Input/1 -> Product9/1
  Delay5/1 -> Product8/2
  Divide1/1 -> Product8/1  "pBSignal"
  MinMax2/1 -> Divide/1, Sum3/2
  TimeConstant/1 -> Divide1/1, Sum3/1
  Product8/1 -> Sum2/2
  Product9/1 -> Sum2/1
  Divide/1 -> Product9/2  "pASignal"
  Sum2/1 -> Output/1, Delay5/1  "lowPassFilteredOutput"
  Sum3/1 -> Divide1/2, Divide/2  "val"

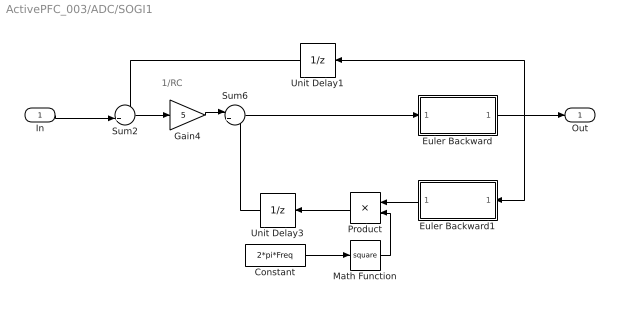
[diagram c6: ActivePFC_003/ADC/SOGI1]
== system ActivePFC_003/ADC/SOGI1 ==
  note: 1/RC
  In : Inport
  Constant : Constant  Value=2*pi*Freq
  Euler Backward : Subsystem  mask{SampleTime=SampleTime, UpperLimit=UpperLimit, LowerLimit=LowerLimit}
      mask prompts: SampleTime "Sample Time"; UpperLimit "Upper Limit"; LowerLimit "Lower Limit"
  Euler Backward1 : Subsystem  mask{SampleTime=SampleTime, UpperLimit=UpperLimit, LowerLimit=LowerLimit}
      mask prompts: SampleTime "Sample Time"; UpperLimit "Upper Limit"; LowerLimit "Lower Limit"
  Gain4 : Gain  Gain=5
  Math Function : Math  Operator=square
  Product : Product
  Sum2 : Sum  Inputs=-+|
  Sum6 : Sum  Inputs=|+-
  Unit Delay1 : UnitDelay  SampleTime=-1
  Unit Delay3 : UnitDelay  SampleTime=-1
  Out : Outport
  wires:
  Unit Delay3/1 -> Sum6/2
  Sum6/1 -> Euler Backward/1(In)
  Euler Backward1/1(Out) -> Product/1
  Constant/1 -> Math Function/1
  Euler Backward/1(Out) -> Euler Backward1/1(In), Out/1, Unit Delay1/1
  In/1 -> Sum2/2
  Product/1 -> Unit Delay3/1
  Sum2/1 -> Gain4/1
  Unit Delay1/1 -> Sum2/1
  Gain4/1 -> Sum6/1
  Math Function/1 -> Product/2

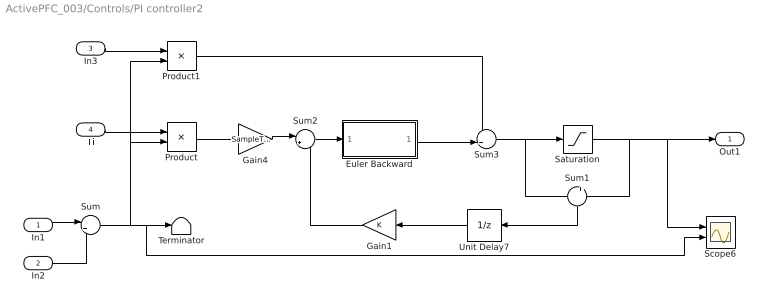
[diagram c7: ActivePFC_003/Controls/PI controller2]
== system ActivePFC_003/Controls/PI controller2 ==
  In1 : Inport
  In2 : Inport  Port=2
  In3 : Inport  Port=3
  Ti : Inport  Port=4
  Euler Backward : Subsystem  mask{SampleTime=SampleTime}
      mask prompts: SampleTime "Sample Time"
  Gain1 : Gain
  Gain4 : Gain  Gain=SampleTime
  Product : Product
  Product1 : Product
  Saturation : Saturate  UpperLimit=UpperLimit  LowerLimit=LowerLimit
  Scope6 : Scope  NumInputPorts=2
  Sum : Sum  Inputs=|+-
  Sum1 : Sum  Inputs=-+
  Sum2 : Sum  Inputs=|++
  Sum3 : Sum  Inputs=++|
  Terminator : Terminator
  Unit Delay7 : UnitDelay  SampleTime=-1
  Out1 : Outport
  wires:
  Unit Delay7/1 -> Gain1/1
  Gain1/1 -> Sum2/2
  Sum1/1 -> Unit Delay7/1
  Sum2/1 -> Euler Backward/1(In)
  Gain4/1 -> Sum2/1
  Euler Backward/1(Out) -> Sum3/2
  Saturation/1 -> Scope6/1, Out1/1, Sum1/2
  Sum/1 -> Product/2, Product1/2, Scope6/2, Terminator/1
  Product/1 -> Gain4/1
  Product1/1 -> Sum3/1
  In2/1 -> Sum/2
  In1/1 -> Sum/1
  In3/1 -> Product1/1
  Sum3/1 -> Saturation/1, Sum1/1
  Ti/1 -> Product/1

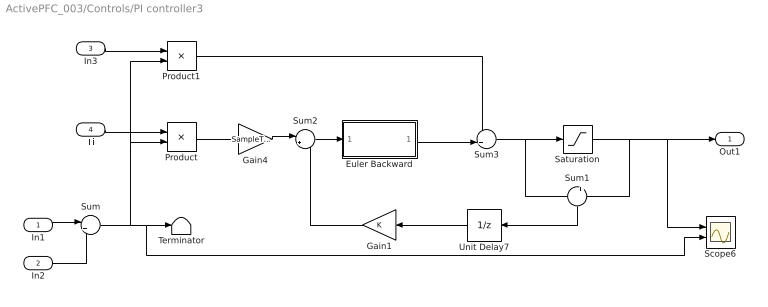
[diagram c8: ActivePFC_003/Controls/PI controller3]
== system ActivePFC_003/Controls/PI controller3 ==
  In1 : Inport
  In2 : Inport  Port=2
  In3 : Inport  Port=3
  Ti : Inport  Port=4
  Euler Backward : Subsystem  mask{SampleTime=SampleTime}
      mask prompts: SampleTime "Sample Time"
  Gain1 : Gain
  Gain4 : Gain  Gain=SampleTime
  Product : Product
  Product1 : Product
  Saturation : Saturate  UpperLimit=UpperLimit  LowerLimit=LowerLimit
  Scope6 : Scope  NumInputPorts=2
  Sum : Sum  Inputs=|+-
  Sum1 : Sum  Inputs=-+
  Sum2 : Sum  Inputs=|++
  Sum3 : Sum  Inputs=++|
  Terminator : Terminator
  Unit Delay7 : UnitDelay  SampleTime=-1
  Out1 : Outport
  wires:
  Ti/1 -> Product/1
  Sum3/1 -> Sum1/1, Saturation/1
  In3/1 -> Product1/1
  In1/1 -> Sum/1
  In2/1 -> Sum/2
  Product1/1 -> Sum3/1
  Product/1 -> Gain4/1
  Sum/1 -> Terminator/1, Scope6/2, Product1/2, Product/2
  Saturation/1 -> Sum1/2, Out1/1, Scope6/1
  Euler Backward/1(Out) -> Sum3/2
  Gain4/1 -> Sum2/1
  Sum2/1 -> Euler Backward/1(In)
  Sum1/1 -> Unit Delay7/1
  Gain1/1 -> Sum2/2
  Unit Delay7/1 -> Gain1/1

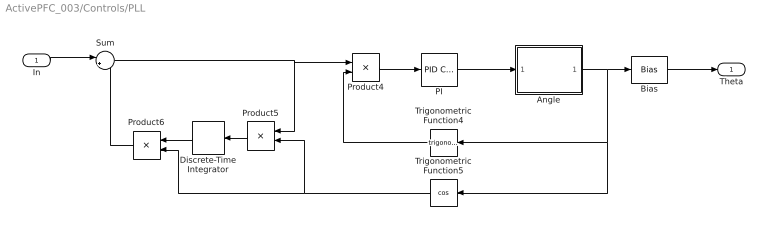
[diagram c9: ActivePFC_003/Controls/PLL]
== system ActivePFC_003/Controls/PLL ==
  In : Inport
  Angle : Subsystem
  Bias : Bias  Bias=-pi/2
  Discrete-Time Integrator : DiscreteIntegrator  gainval=100*2  SampleTime=-1  LimitOutput=on  UpperSaturationLimit=1000  LowerSaturationLimit=-1000  ICPrevOutput=DiscIntNeverNeededParam  ICPrevScaledInput=DiscIntNeverNeededParam
  PI : simulink/Continuous/PID Controller  Controller=PI  TimeDomain=Discrete-time  SampleTime=-1  IntegratorMethod=Forward Euler  FilterMethod=Forward Euler  Form=Parallel  UseFilter=on  ControllerParametersSource=internal  P=4  I=1040  D=0  N=100  InitialConditionSource=internal  InitialConditionForIntegrator=2*pi*60  InitialConditionForFilter=0  ExternalReset=none  LimitOutput=on  UpperSaturationLimit=2*50*pi*1.2  LowerSaturationLimit=-10  LinearizeAsGain=off  AntiWindupMode=none  Kb=1  TrackingMode=off  Kt=1  PParamMin=[]  PParamMax=[]  IParamMin=[]  IParamMax=[]  DParamMin=[]  DParamMax=[]  NParamMin=[]  NParamMax=[]  KbParamMin=[]  KbParamMax=[]  KtParamMin=[]  KtParamMax=[]  POutMin=[]  POutMax=[]  IOutMin=[]  IOutMax=[]  DOutMin=[]  DOutMax=[]  NOutMin=[]  NOutMax=[]  KbOutMin=[]  KbOutMax=[]  KtOutMin=[]  KtOutMax=[]  IntegratorOutMin=[]  IntegratorOutMax=[]  FilterOutMin=[]  FilterOutMax=[]  SumOutMin=[]  SumOutMax=[]  SumI1OutMin=[]  SumI1OutMax=[]  SumI2OutMin=[]  SumI2OutMax=[]  SumI3OutMin=[]  SumI3OutMax=[]  SumDOutMin=[]  SumDOutMax=[]  SaturationOutMin=[]  SaturationOutMax=[]  IntegratorContinuousStateAttributes=''  IntegratorStateMustResolveToSignalObject=off  IntegratorRTWStateStorageClass=Auto  FilterContinuousStateAttributes=''  FilterStateMustResolveToSignalObject=off  FilterRTWStateStorageClass=Auto  DifferentiatorICPrevScaledInput=0  DifferentiatorOutMin=[]  DifferentiatorOutMax=[]  FilterDiffOutCoefMin=[]  FilterDiffOutCoefMax=[]  SumDenOutMin=[]  SumDenOutMax=[]  SumNumOutMin=[]  SumNumOutMax=[]  ReciprocalOutMin=[]  ReciprocalOutMax=[]  DivideOutMin=[]  DivideOutMax=[]  TunerSelectOption=Transfer Function Based (PID Tuner App)
  Product4 : Product
  Product5 : Product
  Product6 : Product
  Sum : Sum  Inputs=|+-
  Trigonometric Function4 : Trigonometry
  Trigonometric Function5 : Trigonometry  Operator=cos
  Theta : Outport
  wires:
  Bias/1 -> Theta/1
  In/1 -> Sum/1
  Trigonometric Function5/1 -> Product6/2, Product5/2
  Product5/1 -> Discrete-Time Integrator/1
  Product6/1 -> Sum/2
  Discrete-Time Integrator/1 -> Product6/1
  Angle/1(theta) -> Bias/1, Trigonometric Function4/1, Trigonometric Function5/1
  Sum/1 -> Product4/1, Product5/1
  Product4/1 -> PI/1
  PI/1 -> Angle/1(omega)
  Trigonometric Function4/1 -> Product4/2

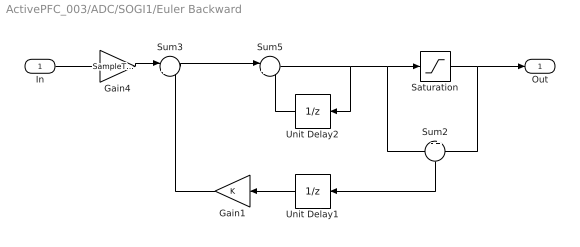
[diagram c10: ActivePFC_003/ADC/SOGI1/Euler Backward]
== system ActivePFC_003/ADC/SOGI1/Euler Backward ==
  In : Inport
  Gain1 : Gain
  Gain4 : Gain  Gain=SampleTime
  Saturation : Saturate  UpperLimit=UpperLimit  LowerLimit=LowerLimit
  Sum2 : Sum  Inputs=-+
  Sum3 : Sum  Inputs=|++
  Sum5 : Sum  Inputs=|++
  Unit Delay1 : UnitDelay  SampleTime=-1
  Unit Delay2 : UnitDelay  SampleTime=-1
  Out : Outport
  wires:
  Sum5/1 -> Saturation/1, Sum2/1, Unit Delay2/1
  Sum2/1 -> Unit Delay1/1
  Gain4/1 -> Sum3/1
  Unit Delay1/1 -> Gain1/1
  In/1 -> Gain4/1
  Saturation/1 -> Out/1, Sum2/2
  Gain1/1 -> Sum3/2
  Sum3/1 -> Sum5/1
  Unit Delay2/1 -> Sum5/2

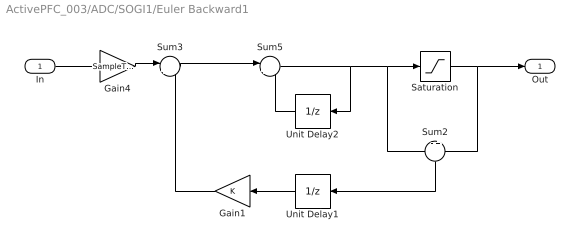
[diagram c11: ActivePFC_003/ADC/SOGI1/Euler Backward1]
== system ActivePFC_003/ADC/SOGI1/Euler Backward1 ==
  In : Inport
  Gain1 : Gain
  Gain4 : Gain  Gain=SampleTime
  Saturation : Saturate  UpperLimit=UpperLimit  LowerLimit=LowerLimit
  Sum2 : Sum  Inputs=-+
  Sum3 : Sum  Inputs=|++
  Sum5 : Sum  Inputs=|++
  Unit Delay1 : UnitDelay  SampleTime=-1
  Unit Delay2 : UnitDelay  SampleTime=-1
  Out : Outport
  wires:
  Unit Delay2/1 -> Sum5/2
  Sum3/1 -> Sum5/1
  Gain1/1 -> Sum3/2
  Saturation/1 -> Sum2/2, Out/1
  In/1 -> Gain4/1
  Unit Delay1/1 -> Gain1/1
  Gain4/1 -> Sum3/1
  Sum2/1 -> Unit Delay1/1
  Sum5/1 -> Unit Delay2/1, Sum2/1, Saturation/1

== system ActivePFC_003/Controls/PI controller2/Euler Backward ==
  In : Inport
  Sum1 : Sum  Inputs=|++
  Unit Delay7 : UnitDelay  SampleTime=-1
  Out : Outport
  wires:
  Sum1/1 -> Unit Delay7/1, Out/1
  Unit Delay7/1 -> Sum1/2
  In/1 -> Sum1/1

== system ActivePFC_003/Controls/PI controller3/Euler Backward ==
  In : Inport
  Sum1 : Sum  Inputs=|++
  Unit Delay7 : UnitDelay  SampleTime=-1
  Out : Outport
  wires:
  In/1 -> Sum1/1
  Unit Delay7/1 -> Sum1/2
  Sum1/1 -> Out/1, Unit Delay7/1

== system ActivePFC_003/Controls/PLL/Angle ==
  omega : Inport
  Add3 : Sum  Inputs=-+
  Constant3 : Constant  Value=2*pi
  Discrete-Time Integrator2 : DiscreteIntegrator  ExternalReset=rising  InitialConditionSource=external  SampleTime=-1  LimitOutput=on  UpperSaturationLimit=10  LowerSaturationLimit=-1  ShowStatePort=on  ICPrevOutput=DiscIntNeverNeededParam  ICPrevScaledInput=DiscIntNeverNeededParam
  Initial : InitialCondition  Value=0
  Relational Operator1 : RelationalOperator  Operator=>  OutDataTypeStr=boolean
  theta : Outport
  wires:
  Add3/1 -> Initial/1
  Initial/1 -> Discrete-Time Integrator2/3
  Relational Operator1/1 -> Discrete-Time Integrator2/2
  Discrete-Time Integrator2/State -> Add3/2, Relational Operator1/1
  Discrete-Time Integrator2/1 -> theta/1
  omega/1 -> Discrete-Time Integrator2/1
  Constant3/1 -> Relational Operator1/2, Add3/1
